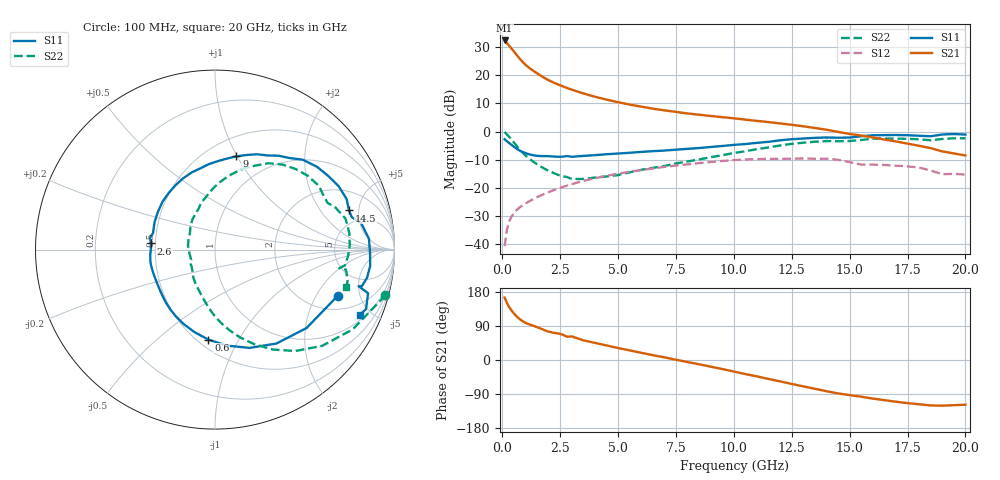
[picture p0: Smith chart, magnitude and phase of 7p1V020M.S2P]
! Infineon Technologies  Discrete & RF Semiconductors
! bfp620
! VCE =  1.0 V,  IC =  20 mA
! Common Emitter S-Parameters:  Sep 2002
# GHz  S  MA  R  50
!  f  S11  S21  S12  S22
! GHz  MAG  ANG  MAG  ANG  MAG  ANG  MAG  ANG
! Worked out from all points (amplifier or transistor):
!   59 points, 100 MHz to 20 GHz, reference 50 ohm
!   highest |S21| = 32.3 dB at 100 MHz (marker M1)
!   |S21| within 3 dB of that: start of sweep to 413 MHz
!   unconditionally stable (mu >= 1): 3.471 GHz to 10.03 GHz; 17.1 GHz to end of sweep
!   at 1 GHz: K = 0.69, MSG = 24.6 dB, |S12| = -25.5 dB
!   at 5.5 GHz: K = 1.04, MAG = 10.7 dB, |S12| = -14.3 dB
!   at 20 GHz: K = 1.40, MAG = -0.4 dB, |S12| = -15.3 dB
!   S11 on the Smith chart (normalised r, x): 100 MHz: 2.82, -3.11; 600 MHz: 0.56, -0.76; 2.6 GHz: 0.47, +0.04; 9 GHz: 0.68, +0.99; 14.5 GHz: 3.53, +3.90; 20 GHz: 1.28, -4.28
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0.1  0.7313 -20.5  41.21 164.7  0.0093 79.5  0.9833 -15.0
0.2  0.6716 -40.6  36.86 150.6  0.0185 71.4  0.8866 -30.1
0.3  0.6253 -56.8  33.14 139.4  0.0256 66.3  0.8026 -41.9
0.4  0.5807 -70.6  29.63 130.4  0.0312 62.3  0.721 -51.6
0.5  0.5389 -83.0  26.34 122.7  0.0359 59.2  0.6429 -60.0
0.6  0.5027 -94.2  23.36 116.2  0.0399 56.8  0.5716 -67.4
0.7  0.4732 -104.2  20.78 110.5  0.0435 55.1  0.5093 -74.0
0.8  0.4496 -113.0  18.6 105.7  0.0468 54.0  0.4567 -79.8
0.9  0.4307 -120.6  16.8 101.7  0.05 53.2  0.4131 -84.9
1.1  0.4022 -132.8  14.12 95.6  0.0561 52.4  0.3472 -93.2
1.4  0.3764 -146.9  11.49 89.0  0.0653 51.5  0.281 -103.3
1.8  0.3673 -163.0  9.05 79.3  0.078 49.9  0.2223 -118.3
2.6  0.3588 174.5  6.372 67.0  0.104 45.4  0.1611 -144.2
3.5  0.3704 155.2  4.742 52.0  0.1333 38.3  0.1443 -172.7
5  0.4079 129.0  3.315 31.6  0.1795 24.8  0.1695 145.2
7  0.4605 100.0  2.376 7.0  0.2362 5.7  0.2448 112.0
9  0.533 77.1  1.889 -17.6  0.2885 -15.2  0.3514 90.1
10.5  0.6008 60.8  1.629 -37.2  0.3201 -33.4  0.4486 74.7
13.5  0.7742 27.1  1.159 -75.9  0.3309 -68.7  0.6602 38.6
14.5  0.7779 16.3  0.987 -88.2  0.3164 -83.8  0.6754 26.2
17  0.8694 -6.0  0.668 -110.1  0.2487 -99.9  0.7512 1.8
20  0.8848 -24.3  0.377 -118.0  0.1727 -110.7  0.7607 -15.9
